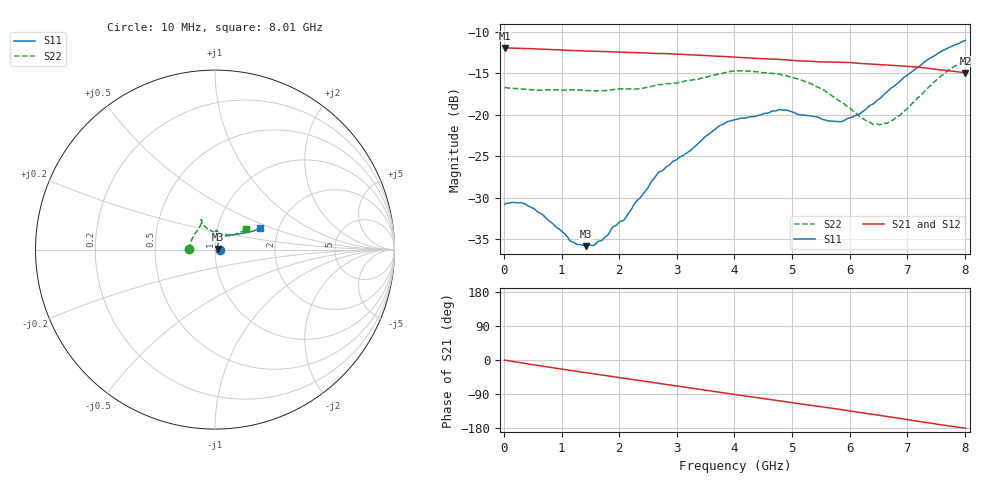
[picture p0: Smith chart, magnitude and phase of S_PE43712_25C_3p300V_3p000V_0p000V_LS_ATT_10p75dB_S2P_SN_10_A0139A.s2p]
! DEVICE ID: PE43712
! File Path: z:\PE43713\PE43713_CHAR_NOM_04292014\AMB\3p300\LS_ATT_10p75dB\PE43713_AMB_3p300V_3p000V_0p000V_LS_ATT_10p75dB_S2P_SN_10_A0139A.s2p
! Serial: 10
! Lot: A0139A
! Temp: 25C
! VDD: 3.300
! VSS: 0.000
! Control_Hi: 3.000
! Control_Lo: 0.000
! Attenuation Step: 10.75dB
! Port 1: RF1
! Port 2: RF2
! ThroughPath:1-2
! IDD: 0.0001467469
! ISS: -1.594e-007
#  Hz  S  RI  R  50
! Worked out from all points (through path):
!   801 points, 10 MHz to 8.01 GHz, reference 50 ohm
!   highest |S21| = -11.93 dB at 10 MHz (marker M1); lowest = -14.9 dB at 8.01 GHz (marker M2)
!   group delay of S21, straight-line fit = 61.8 ps
!   lowest |S11| = -35.8 dB at 1.42 GHz (marker M3), VSWR 1.03, Z = 51.6 + j0.408 ohm
!   |S11| at or under -10 dB: start of sweep to end of sweep
!   |S22| runs from -21.2 to -13.6 dB; largest |S21 - S12| = 0.00091
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1e7  0.0289 0.000145  0.2531 -0.00133  0.2532 -0.0013  -0.1462 0.00091
3.7e8  0.0289 -0.00331  0.2476 -0.0399  0.2485 -0.0401  -0.1418 0.0171
6.8e8  0.0246 -0.00366  0.2379 -0.071  0.238 -0.0711  -0.1372 0.0317
1.17e9  0.0173 0.000719  0.2159 -0.1138  0.2159 -0.1139  -0.1313 0.0526
1.35e9  0.0162 0.00289  0.2065 -0.128  0.2065 -0.1281  -0.1276 0.0591
1.42e9  0.0157 0.00396  0.2025 -0.1334  0.2025 -0.1334  -0.1255 0.0624
1.7e9  0.0145 0.00986  0.1855 -0.1534  0.1855 -0.1534  -0.1182 0.0747
1.89e9  0.0149 0.015  0.1728 -0.1659  0.1728 -0.1659  -0.1138 0.0845
2.09e9  0.014 0.0187  0.1586 -0.178  0.1586 -0.178  -0.11 0.0918
2.68e9  0.0194 0.0406  0.1119 -0.2054  0.1118 -0.2054  -0.0885 0.1236
3.72e9  0.0142 0.0836  0.0209 -0.2243  0.0207 -0.2243  -0.0749 0.159
4.01e9  0.0113 0.0929  -0.00438 -0.2226  -0.00439 -0.2226  -0.0779 0.1664
4.79e9  0.00706 0.1073  -0.0669 -0.2048  -0.0669 -0.2049  -0.0752 0.1583
5.35e9  0.0175 0.0965  -0.1051 -0.1815  -0.105 -0.1814  -0.0665 0.1374
5.88e9  0.0398 0.0826  -0.1376 -0.1549  -0.1373 -0.1549  -0.0338 0.1129
6.17e9  0.0603 0.0812  -0.1524 -0.1358  -0.1521 -0.1359  -0.00854 0.0974
6.39e9  0.0809 0.0825  -0.1615 -0.1212  -0.1612 -0.1211  0.013 0.0873
6.68e9  0.113 0.0841  -0.1718 -0.1003  -0.1716 -0.1004  0.0447 0.0783
6.88e9  0.1346 0.0864  -0.1778 -0.0854  -0.1776 -0.0854  0.0641 0.0767
7.36e9  0.191 0.0991  -0.1846 -0.0471  -0.1844 -0.0472  0.116 0.0873
7.72e9  0.229 0.1095  -0.1831 -0.02  -0.183 -0.0202  0.1553 0.103
8.01e9  0.253 0.121  -0.179 -0.000951  -0.1787 -0.00122  0.1754 0.1138
